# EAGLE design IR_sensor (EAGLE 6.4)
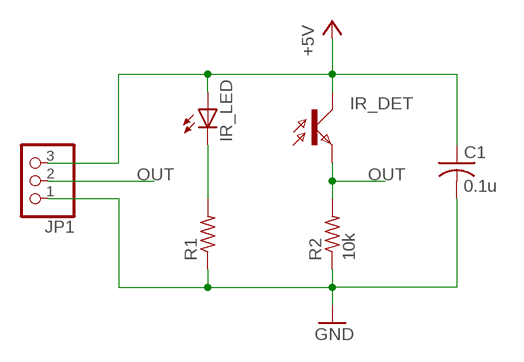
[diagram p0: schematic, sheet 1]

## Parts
C1  0.1u  C-US025-030X050  [C025-030X050]
IR_DET  BPX81  [BPX81]
IR_LED  LED5MM  [LED5MM]
JP1  PINHD-1X3  [1X03]
R1  R-US_0204/7  [0204/7]
R2  10k  R-US_0204/7  [0204/7]

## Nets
+5V: C1.1 IR_DET.C IR_LED.A JP1.3
GND: C1.2 JP1.1 R1.1 R2.1
N$2: IR_LED.K(C) R1.2
OUT: IR_DET.E JP1.2 R2.2

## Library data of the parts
C1 = rcl:C-US: CAPACITOR, American symbol
IR_DET = opto-trans-siemens:BPX81: PHOTO TRANSISTOR; OC_FARNELL: unknown; OC_NEWARK: unknown
IR_LED = led:LED: LED
JP1 = pinhead:PINHD-1X3: PIN HEADER
R1 R2 = rcl:R-US_: RESISTOR, American symbol

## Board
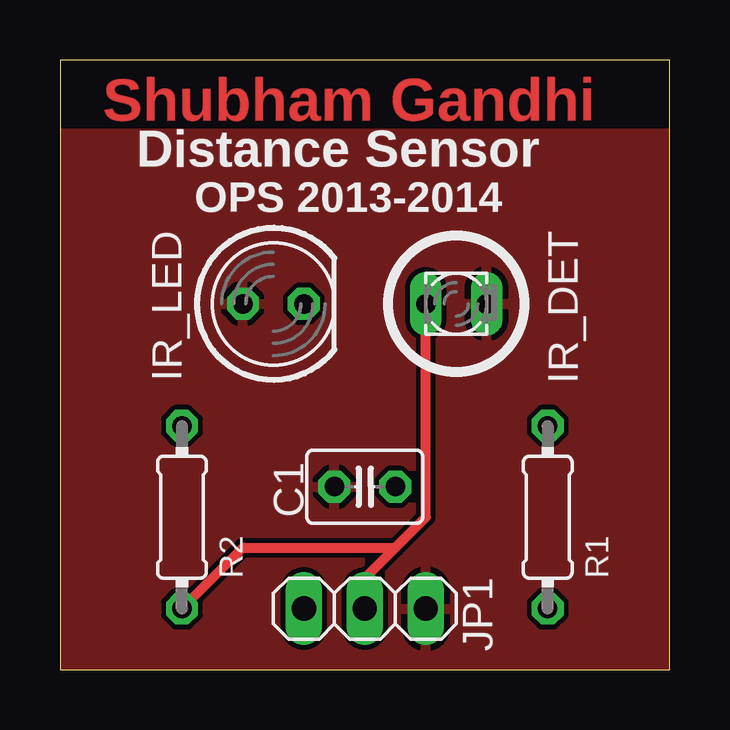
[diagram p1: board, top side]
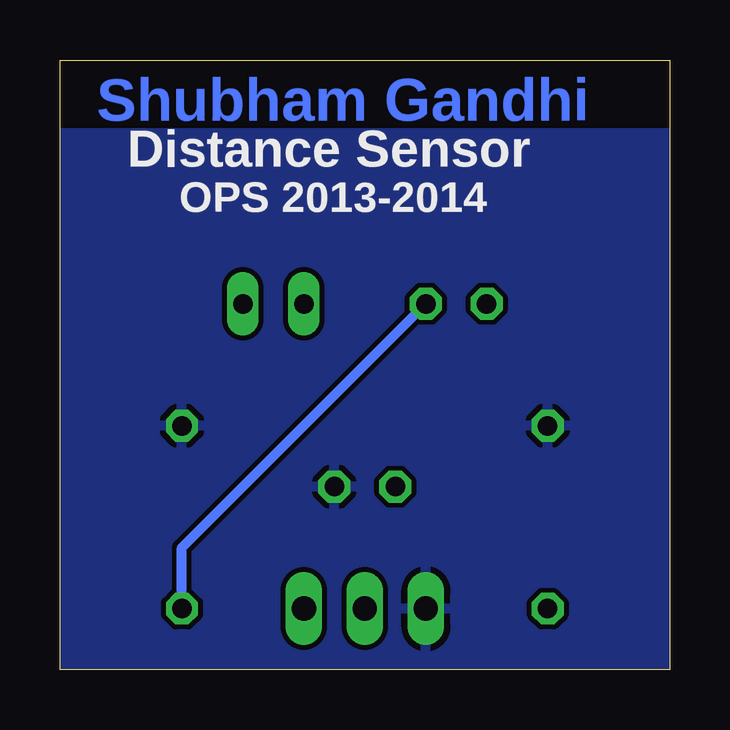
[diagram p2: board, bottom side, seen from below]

Size 25.4 x 25.4 mm. Coordinates in mm from the lower left corner, seen from the top.
Outline: 0,0 25.4,0 25.4,25.4 0,25.4 0,0
Copper layers (1*16): Top 0.035mm / dielectric 1.5mm / Bottom 0.035mm
Design rules "default *": minimum track width 10mil, minimum drill 24mil, track to track 8mil, track to pad 8mil, pad to pad 8mil, via to via 8mil, smd to smd 8mil, copper to edge 1mil, drill to drill 8mil, minimum pad ring 10mil, minimum via ring 8mil, stop-mask expansion 4mil, vias tented up to drill 0mil, thermal gap 10mil

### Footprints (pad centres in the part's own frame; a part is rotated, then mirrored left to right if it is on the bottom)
C025-030X050 = drill 0.813 octagon: 1 -1.27,0; 2 1.27,0
BPX81 = drill 0.813 long: C 1.27,0; E -1.27,0
LED5MM = drill 0.813 octagon: A -1.27,0; K 1.27,0
1X03 = drill 1.016 long: 1 -2.54,0; 2 0,0; 3 2.54,0
0204/7 = drill 0.813 octagon: 1 -3.81,0; 2 3.81,0

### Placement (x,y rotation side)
C1  12.7,7.62 0 top
IR_DET  16.51,15.24 0 top
IR_LED  8.89,15.24 0 top
JP1  12.7,2.54 0 top
R1  20.32,6.35 270 top
R2  5.08,6.35 270 top

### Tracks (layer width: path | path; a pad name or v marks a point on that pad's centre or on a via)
+5V
  pour Top: 0,0 0,22.35 25.4,22.35 25.4,0
GND
  pour Bottom: 0,0 0,22.35 25.4,22.35 25.4,0
N$2
  Bottom 0.406: R1.2 20.32,5.08 IR_LED.K
OUT
  Top 0.406: JP1.2 12.7,3.81 13.97,5.08 | 13.97,5.08 15.24,6.35 IR_DET.E | R2.2 7.62,5.08 13.97,5.08

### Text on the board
Top: Shubham Gandhi
Bottom: Shubham Gandhi
tPlace: Distance Sensor | OPS 2013-2014
bPlace: Distance Sensor | OPS 2013-2014
tStop: Shubham Gandhi
bStop: Shubham Gandhi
